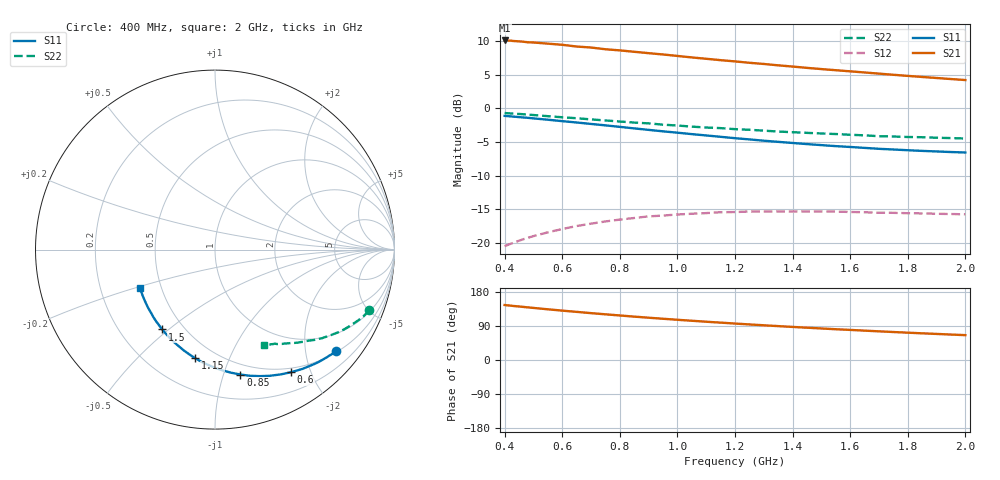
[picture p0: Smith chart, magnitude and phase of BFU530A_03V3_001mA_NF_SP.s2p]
! Filename:  P:\Prog\Test\Noise\ATS_data\Testdata_Net\06 Compressed Noise after Statistics\BFU530A_APG2013_33_A05_03p3V_001mA_SP_CM01_D.sf
! Date/Time: Tue 16/Apr/2013 15:10:54
! BFU530A_APG2013_33_A05_03p3V_1to25mA_NF_CM01_Bias1_R.sf
! Noise Parameter Data File
! BFU530A_APG2013_33_A05_03p3V_1to25mA_NF_CM01
! Date/time: Fri Apr 12 14:21:19 2013
! freq range =  0.4000 to  2.0000 GHz, 37 points
! bias range =  1.0000 to 24.9950 mA, 8 points
! bias supplies used: 1 1 0 0 0 0
! VAR bias_mode= 1  ! Specify V_out, I_out
! VAR bias_var = 1  ! Bias variable = I_out
! VAR V_out= 3.300000
! VAR I_out= 1.000000
! VAR V_in= 0.784200
! VAR I_in= 0.010501
! Device data file deembeded for feedlines and parallel
! Original file: \06 Compressed Noise after Statistics\BFU530A_APG2013_33_A05_03p3V_001mA_SP_CM01_R.sf
! Feed-files: PR017V01_150413_Feed1.s2p, PR017V01_150413_Feed2.s2p
! Parallel-file: PR017V01_150413_Par.s2p
# MHz S MA R 50
!  Freq-MHz  S11-mag  S11-arg  S21-mag  S21-arg  S12-mag  S12-arg  S22-mag  S22-arg
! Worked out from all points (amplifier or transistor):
!   37 points, 400 MHz to 2 GHz, reference 50 ohm
!   highest |S21| = 10.1 dB at 400 MHz (marker M1)
!   |S21| within 3 dB of that: start of sweep to 1.168 GHz
!   unconditionally stable (mu >= 1): nowhere
!   at 500 MHz: K = 0.23, MSG = 14.4 dB, |S12| = -19.0 dB
!   at 1.1 GHz: K = 0.48, MSG = 11.5 dB, |S12| = -15.6 dB
!   at 2 GHz: K = 0.88, MSG = 10.0 dB, |S12| = -15.8 dB
!   lowest NFmin = 0.53 dB at 420 MHz
!   S11 on the Smith chart (normalised r, x): 400 MHz: 0.53, -2.66; 600 MHz: 0.44, -1.71; 850 MHz: 0.41, -1.14; 1.15 GHz: 0.39, -0.76; 1.5 GHz: 0.38, -0.48; 2 GHz: 0.38, -0.21
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400  0.88 -40.0  3.202 145.1  0.09446 64.8  0.924 -21.5
420  0.873 -41.9  3.192 143.4  0.09825 63.7  0.9177 -22.4
460  0.858 -45.6  3.142 140.4  0.1055 61.6  0.9065 -24.2
480  0.8515 -47.4  3.105 138.9  0.1089 60.6  0.8994 -25.1
500  0.8432 -49.2  3.093 137.4  0.1122 59.6  0.8929 -26.0
550  0.824 -53.8  3.032 133.8  0.1197 57.2  0.8754 -28.0
600  0.804 -58.2  2.974 130.3  0.1267 54.9  0.8594 -30.0
650  0.7858 -62.2  2.886 127.0  0.1334 52.8  0.8452 -31.8
700  0.7665 -66.6  2.837 123.7  0.1389 50.8  0.8286 -33.6
750  0.748 -70.5  2.755 120.6  0.1443 48.9  0.8137 -35.2
800  0.7291 -74.6  2.701 117.5  0.1489 47.1  0.799 -36.8
850  0.7101 -78.5  2.638 114.5  0.153 45.4  0.7845 -38.4
950  0.6753 -86.2  2.519 108.8  0.1595 42.3  0.7571 -41.3
1050  0.6438 -93.3  2.395 103.5  0.1646 39.7  0.7322 -43.8
1150  0.6148 -100.5  2.285 98.6  0.169 37.3  0.7134 -46.0
1200  0.6006 -103.9  2.236 96.2  0.1694 36.3  0.701 -47.3
1350  0.564 -113.8  2.091 89.4  0.1711 33.9  0.6729 -50.6
1500  0.5333 -123.5  1.961 83.2  0.1711 32.2  0.6509 -53.6
1650  0.5086 -132.6  1.851 77.5  0.1689 31.5  0.6303 -56.6
1750  0.4948 -138.6  1.779 73.9  0.1672 31.6  0.6183 -58.4
1850  0.4831 -144.4  1.714 70.4  0.1656 31.9  0.6105 -60.2
2000  0.4699 -152.9  1.626 65.6  0.1629 33.4  0.5972 -63.0
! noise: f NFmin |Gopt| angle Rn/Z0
400  0.5465  0.6285  23.39  0.3403
460  0.5893  0.6258  26.96  0.356
600  0.7169  0.577  34.67  0.3218
800  0.6627  0.5732  50.82  0.2593
1000  0.6705  0.5739  63.58  0.2406
1200  0.8334  0.5695  76.44  0.2241
1400  0.8257  0.5739  90.89  0.1798
1600  0.913  0.4975  106.9  0.1425
1800  0.7441  0.4985  121.5  0.1031
2000  0.8427  0.4946  133.1  0.095
